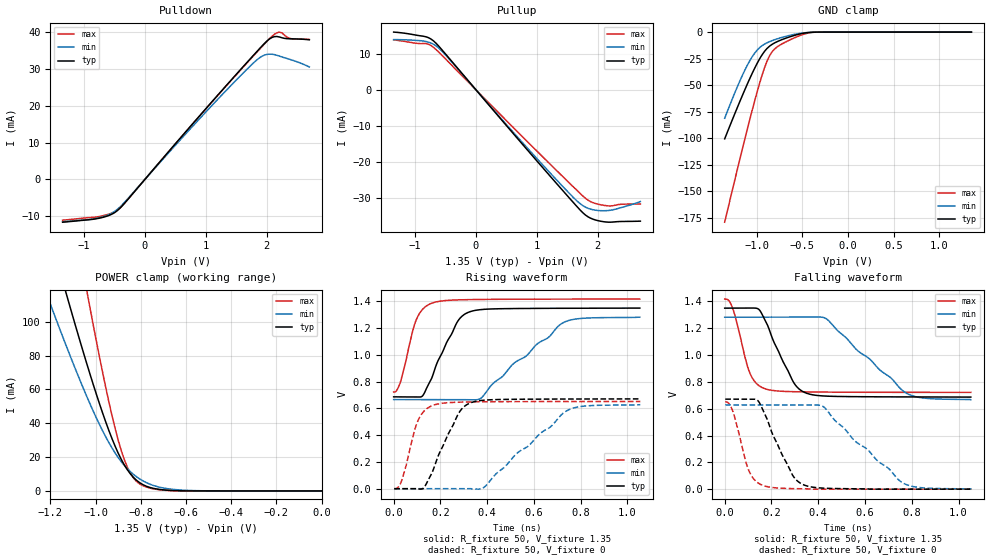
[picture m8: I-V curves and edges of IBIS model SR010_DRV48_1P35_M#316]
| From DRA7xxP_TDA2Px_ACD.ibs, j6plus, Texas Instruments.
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| Model based on original model for DDR_DIFFIOPB_V
|   Sub model SR010_DRV48_1P35
[model]   SR010_DRV48_1P35_M#316
|[Description]  [1.35V-I/O-X-X]
|   , ,
|[Input Load]
|[Output Drive]
|Voltage   1.35V
|Mode   I/O
Model_type   I/O
Polarity   Non-Inverting
Enable   Active-Low
Vinl =  0.585
Vinh =  0.765
Cref =  15.0000pF
Rref =  100.0000M
Vref =  0V
Vmeas =  0.675
C_comp   2p   2p   2p
[Model Spec]
Vinl   0.585   0.55125   0.61875
Vinh   0.765   0.73125   0.79875
[Receiver Thresholds]
Tslew_ac = 5n
Vth = 0.675
Vth_max = 0.709
Vth_min = 0.608
Vinh_ac = 0.175
Vinh_dc = 0.1
Vinl_ac = -0.175
Vinl_dc = -0.1
[Temperature Range]   25   125   -40
[Voltage Range]   1.35   1.2825   1.4175
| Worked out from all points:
|   slope of the pulldown table from 0 to 0.203 V, typ, clamps not added: 51.5 ohm
|   slope of the pullup table from 0 to 0.203 V, typ, clamps not added: 50.4 ohm
|   GND clamp passes 1 mA (typ) near -0.48 V on its own axis
|   POWER clamp passes 1 mA (typ) near -0.72 V on its own axis
|   rising waveform, R_fixture 50, V_fixture 1.35: 20-80 % time 102ps typ, 250ps min, 62.1ps max; typ from 0.687 V to 1.35 V
|   rising waveform, R_fixture 50, V_fixture 0: 20-80 % time 102ps typ, 245ps min, 60.9ps max; typ from 0 V to 0.671 V
|   falling waveform, R_fixture 50, V_fixture 1.35: 20-80 % time 103ps typ, 233ps min, 62.5ps max; typ from 1.35 V to 0.687 V
|   falling waveform, R_fixture 50, V_fixture 0: 20-80 % time 103ps typ, 239ps min, 60.1ps max; typ from 0.671 V to 0 V
[POWER_clamp]
-1.35V    224.4mA    165.8mA    358.5mA
-1.214V   157mA      115.5mA    250.8mA
-1.132V   117.8mA    86.59mA    187.7mA
-1.118V   111.4mA    81.92mA    177.3mA
-1.036V   74.26mA    55.16mA    116.8mA
-954.5mV  40.7mA     31.91mA    61.06mA
-900mV    22.42mA    19.79mA    30.14mA
-859.1mV  12.48mA    13.09mA    13.96mA
-804.5mV  4.85mA     7.084mA    4.132mA
-736.4mV  1.313mA    2.9mA      1.073mA
-627.3mV  101.6uA    577.3uA    45.9uA
0V        75.63nA    322.4nA    418.5nA
[Pulldown]
-1.35V    -11.61mA   -11.5mA    -11.06mA
-736.4mV  -10.48mA   -10.33mA   -10.03mA
-531.8mV  -9.35mA    -9.062mA   -9.043mA
-409.1mV  -7.817mA   -7.49mA    -7.751mA
1.145V    21.94mA    20.88mA    21.88mA
1.718V    32.55mA    30.62mA    32.41mA
1.923V    36.25mA    33.48mA    36.08mA
2.005V    37.61mA    33.98mA    37.53mA
2.086V    38.57mA    34.03mA    38.89mA
2.209V    38.7mA     33.51mA    40.04mA
2.373V    38.22mA    32.66mA    38.36mA
2.7V      37.95mA    30.56mA    38.05mA
[Pullup]
-1.35V    15.95mA    13.86mA    13.81mA
-981.8mV  15.11mA    13.66mA    12.86mA
-818.2mV  14.65mA    13.35mA    12.79mA
-736.4mV  14.02mA    12.92mA    12.23mA
-613.6mV  12.13mA    11.6mA     10.47mA
1.064V    -20.91mA   -20.19mA   -18.01mA
1.555V    -30.35mA   -29.03mA   -26.14mA
1.759V    -34.1mA    -32.12mA   -29.45mA
1.923V    -35.82mA   -33.22mA   -31.26mA
2.168V    -36.64mA   -33.43mA   -32.13mA
2.414V    -36.45mA   -32.48mA   -31.67mA
2.7V      -36.37mA   -30.94mA   -31.63mA
[GND_clamp]
-1.35V    -100.7mA   -81.27mA   -179.3mA
-1.241V   -77.31mA   -57.61mA   -140mA
-1.132V   -54.83mA   -36.31mA   -101.6mA
-1.05V    -39.08mA   -23.36mA   -74mA
-968.2mV  -25.28mA   -14.71mA   -48.34mA
-913.6mV  -18.13mA   -11.32mA   -33.52mA
-859.1mV  -13.28mA   -9.024mA   -22.35mA
-831.8mV  -11.61mA   -8.091mA   -18.64mA
-777.3mV  -9.078mA   -6.444mA   -14.07mA
-531.8mV  -1.871mA   -1.307mA   -3.441mA
-368.2mV  -88.76uA   -111.2uA   -158uA
1.35V     75.63nA    385.5nA    349.4nA
[Ramp]
dV/dt_f 0.39855472/0.10304333n 0.37078817/0.23397463n 0.41787418/62.527126p
dV/dt_r 0.40480031/0.10261282n  0.3790613/0.2464487n 0.39255068/61.058552p
R_load = 50
[Rising Waveform]
R_fixture = 50
V_fixture = 1.35
V_fixture_min = 1.2825
V_fixture_max = 1.4175
0s        686.6mV    666.1mV    722.7mV
29.08ps   685.9mV    666mV      797.2mV
97.74ps   685.1mV    666mV      1.267V
124.6ps   696mV      666mV      1.342V
160.2ps   815.7mV    666.1mV    1.385V
270.2ps   1.241V     665.9mV    1.411V
325.4ps   1.322V     664.5mV    1.413V
374.5ps   1.339V     678.2mV    1.415V
728.4ps   1.349V     1.244V     1.417V
1.053ns   1.35V      1.282V     1.417V
[Rising Waveform]
R_fixture = 50
V_fixture = 0
V_fixture_min = 0
V_fixture_max = 0
2.416ps   0V         0V         0V
33.78ps   0V         0V         57.56mV
106.1ps   -2.582mV   0V         516.9mV
131.3ps   12.29mV    0V         582.5mV
170.7ps   147.8mV    0V         624.7mV
277.3ps   561.9mV    0V         646.8mV
335.4ps   645.8mV    -2.186mV   648.9mV
388.7ps   662mV      13.2mV     649.9mV
746.5ps   670.4mV    588.3mV    651.7mV
1.055ns   671.4mV    628.3mV    651.8mV
[Falling Waveform]
R_fixture = 50
V_fixture = 1.35
V_fixture_min = 1.2825
V_fixture_max = 1.4175
0s        1.35V      1.282V     1.417V
37.02ps   1.35V      1.283V     1.334V
108.9ps   1.35V      1.283V     860.8mV
145ps     1.342V     1.283V     774mV
171ps     1.265V     1.283V     749.8mV
292ps     804.3mV    1.282V     727mV
348.1ps   716.7mV    1.282V     725.2mV
437ps     693.7mV    1.268V     723.7mV
784.8ps   687.8mV    708.7mV    722mV
1.053ns   686.6mV    666.1mV    721.8mV
[Falling Waveform]
R_fixture = 50
V_fixture = 0
V_fixture_min = 0
V_fixture_max = 0
2.416ps   671.4mV    628.3mV    650.8mV
36.33ps   671.6mV    628.3mV    573mV
105.3ps   671.3mV    628.4mV    130.1mV
140.7ps   662.1mV    628.4mV    48.9mV
164.5ps   586.6mV    628.3mV    27.28mV
287.7ps   111.9mV    628.3mV    4.161mV
341.9ps   29.45mV    628.2mV    2.503mV
425ps     7.305mV    611.3mV    0V
765.2ps   0V         43.21mV    0V
1.055ns   0V         0V         0V
